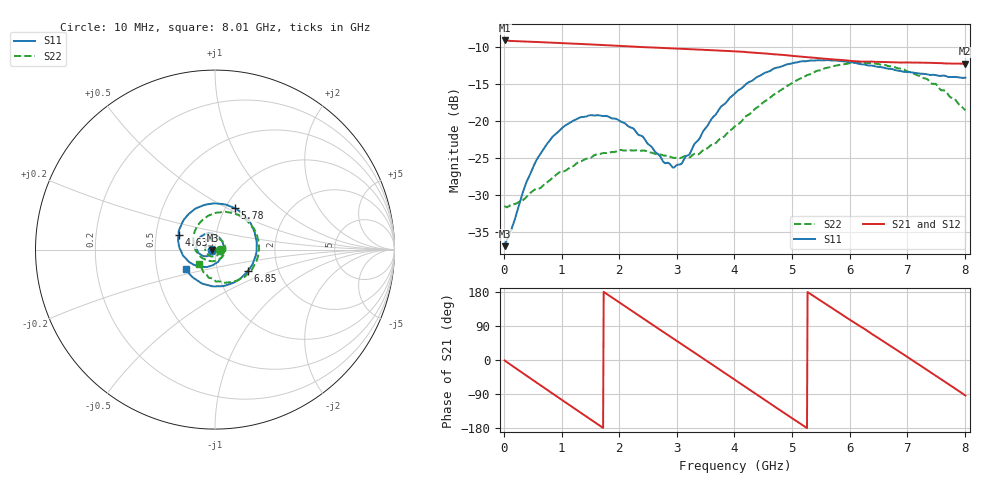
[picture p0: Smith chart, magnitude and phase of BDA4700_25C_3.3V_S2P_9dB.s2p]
!Agilent Technologies,E5071B,MY42404982,A.09.10
!Date: Mon Oct 20 18:06:47 2025
!Data & Calibration Information:
!Freq	S11:SOLT2(ON)	S21:SOLT2(ON)	S12:SOLT2(ON)	S22:SOLT2(ON)
# Hz S RI R 50
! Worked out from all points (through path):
!   801 points, 10 MHz to 8.01 GHz, reference 50 ohm
!   highest |S21| = -9.12 dB at 10 MHz (marker M1); lowest = -12.3 dB at 8 GHz (marker M2)
!   group delay of S21, straight-line fit = 281 ps
!   lowest |S11| = -36.9 dB at 10 MHz (marker M3), VSWR 1.03, Z = 48.6 - j0.147 ohm
!   |S11| at or under -10 dB: start of sweep to end of sweep
!   |S22| runs from -31.7 to -12.1 dB; largest |S21 - S12| = 0.004
!   S11 on the Smith chart (normalised r, x): 10 MHz: 0.97, -0.00; 4.63 GHz: 0.66, +0.11; 5.78 GHz: 1.11, +0.55; 6.85 GHz: 1.40, -0.35; 8.01 GHz: 0.70, -0.16
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1e7  -0.0141 -0.00152  0.3498 -0.00755  0.3498 -0.00777  0.0266 -0.00139
5.9e8  -0.0431 -0.0366  0.1592 -0.302  0.1591 -0.3021  0.00945 -0.0335
9.6e8  -0.0816 -0.0267  -0.0621 -0.3306  -0.0621 -0.3308  -0.0254 -0.037
1.35e9  -0.1048 0.0163  -0.2575 -0.2082  -0.2576 -0.2084  -0.0533 -0.00428
1.93e9  -0.0597 0.0845  -0.3016 0.1144  -0.3017 0.1144  -0.0237 0.057
2.32e9  -4.8e-05 0.0814  -0.1556 0.276  -0.1557 0.2759  0.0261 0.0575
2.68e9  0.0423 0.0415  0.0392 0.3099  0.0388 0.3098  0.0561 0.0193
2.96e9  0.048 -0.0081  0.1796 0.2509  0.1794 0.2504  0.0531 -0.0181
3.37e9  0.00887 -0.0733  0.2962 0.0671  0.2966 0.0671  0.0127 -0.058
3.68e9  -0.0554 -0.0961  0.2837 -0.0964  0.2838 -0.0973  -0.0352 -0.0616
4.01e9  -0.1336 -0.0755  0.1799 -0.2346  0.1802 -0.2342  -0.0845 -0.0362
4.32e9  -0.1881 -0.0106  0.0299 -0.288  0.0298 -0.289  -0.1155 0.0167
4.63e9  -0.2024 0.0824  -0.1236 -0.2552  -0.1231 -0.2556  -0.1165 0.0865
5e9  -0.1528 0.192  -0.246 -0.1235  -0.2468 -0.1243  -0.0666 0.1676
5.35e9  -0.045 0.2518  -0.265 0.0408  -0.2653 0.0392  0.0272 0.2073
5.78e9  0.1118 0.23  -0.1615 0.203  -0.1608 0.203  0.1595 0.175
6.21e9  0.2159 0.1086  0.0154 0.2513  0.0189 0.2516  0.2397 0.0559
6.68e9  0.216 -0.0644  0.1913 0.1598  0.1916 0.1595  0.2155 -0.0926
6.85e9  0.1835 -0.1191  0.228 0.0978  0.2286 0.0961  0.1813 -0.1352
7.36e9  0.0253 -0.2042  0.2184 -0.1156  0.2185 -0.1156  0.0455 -0.1845
8e9  -0.1614 -0.111  -0.0114 -0.2432  -0.0109 -0.2435  -0.0854 -0.0826
8.01e9  -0.1632 -0.1087  -0.0158 -0.243  -0.0151 -0.2433  -0.0864 -0.0802
